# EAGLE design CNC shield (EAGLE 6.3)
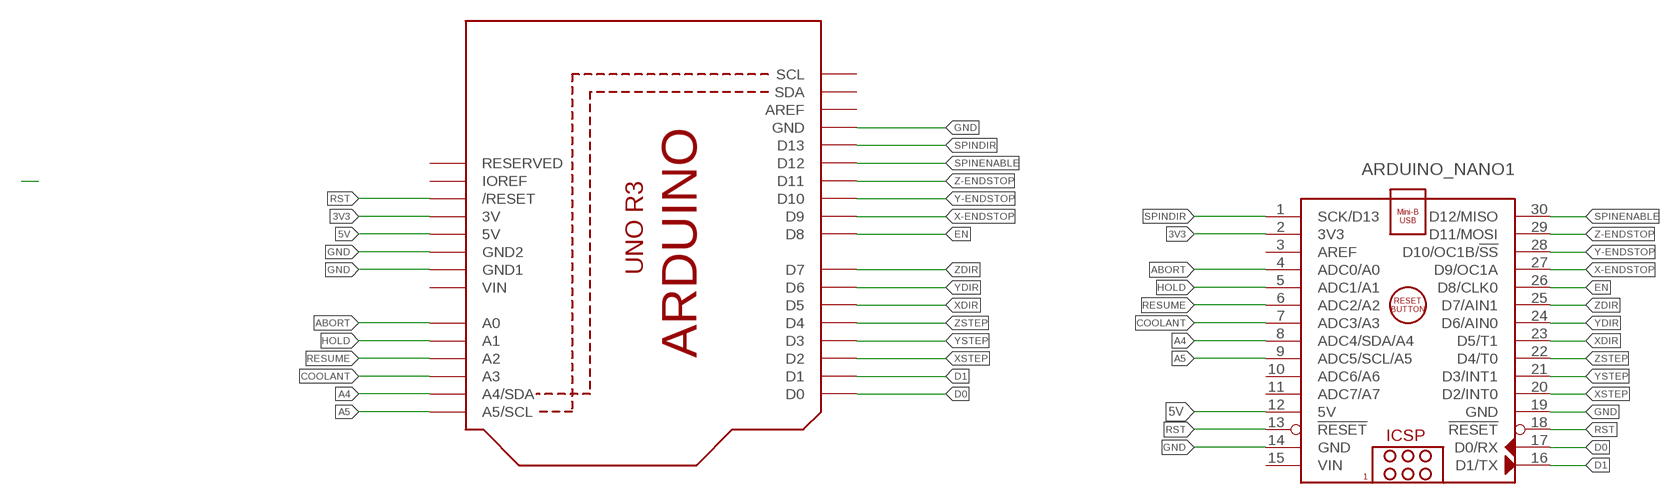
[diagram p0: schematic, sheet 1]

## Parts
ARDUINO_NANO1  ARDUINO_NANO  [ARDUINO_NANO]
U1  ARDUINOR3-BPLACE  [ARDUINOR3-BPLACE]

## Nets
3V3: ARDUINO_NANO1.2(3V3) U1.3V
5V: ARDUINO_NANO1.12(5V) U1.5V
A4: ARDUINO_NANO1.8(ADC4/SDA/A4) U1.A4(A4/SDA)
A5: ARDUINO_NANO1.9(ADC5/SCL/A5) U1.A5(A5/SCL)
ABORT: ARDUINO_NANO1.4(ADC0/A0) U1.A0
COOLANT: ARDUINO_NANO1.7(ADC3/A3) U1.A3
D0: ARDUINO_NANO1.17(D0/RX) U1.D0
D1: ARDUINO_NANO1.16(D1/TX) U1.D1
EN: ARDUINO_NANO1.26(D8/CLK0) U1.D8
GND: ARDUINO_NANO1.14(GND) ARDUINO_NANO1.19(GND) U1.GND U1.GND1 U1.GND2
HOLD: ARDUINO_NANO1.5(ADC1/A1) U1.A1
RESUME: ARDUINO_NANO1.6(ADC2/A2) U1.A2
RST: ARDUINO_NANO1.13(!RESET) ARDUINO_NANO1.18(!RESET) U1.RESET(/RESET)
SPINDIR: ARDUINO_NANO1.1(SCK/D13) U1.D13
SPINENABLE: ARDUINO_NANO1.30(D12/MISO) U1.D12
X-ENDSTOP: ARDUINO_NANO1.27(D9/OC1A) U1.D9
XDIR: ARDUINO_NANO1.23(D5/T1) U1.D5
XSTEP: ARDUINO_NANO1.20(D2/INT0) U1.D2
Y-ENDSTOP: ARDUINO_NANO1.28(D10/OC1B/!SS) U1.D10
YDIR: ARDUINO_NANO1.24(D6/AIN0) U1.D6
YSTEP: ARDUINO_NANO1.21(D3/INT1) U1.D3
Z-ENDSTOP: ARDUINO_NANO1.29(D11/MOSI) U1.D11
ZDIR: ARDUINO_NANO1.25(D7/AIN1) U1.D7
ZSTEP: ARDUINO_NANO1.22(D4/T0) U1.D4
Unconnected: ARDUINO_NANO1.3(AREF) ARDUINO_NANO1.10(ADC6/A6) ARDUINO_NANO1.11(ADC7/A7) U1.AREF U1.IOREF U1.RESERVED U1.SCL U1.SDA

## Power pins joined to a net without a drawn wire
VIN: ARDUINO_NANO1.15(VIN) U1.VIN

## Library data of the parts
ARDUINO_NANO1 = ArduinoNanoV30:ARDUINO_NANO: Arduino Nano V3.0 Module Overview: The Arduino Nano is a small, complete, and breadboard-friendly board based on the ATmega328 (Arduino Nano 3.x) or ATmega168 (Arduino Nano 2.x). It has more or less the same functionality of the Arduino Duemilanove, but in a different package. It lacks only a DC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
U1 = adafruit:ARDUINOR3: This is a new object for the new Arduino R3 - with extra pins that you may want to use (such as IOref, and duplicated A4/A5

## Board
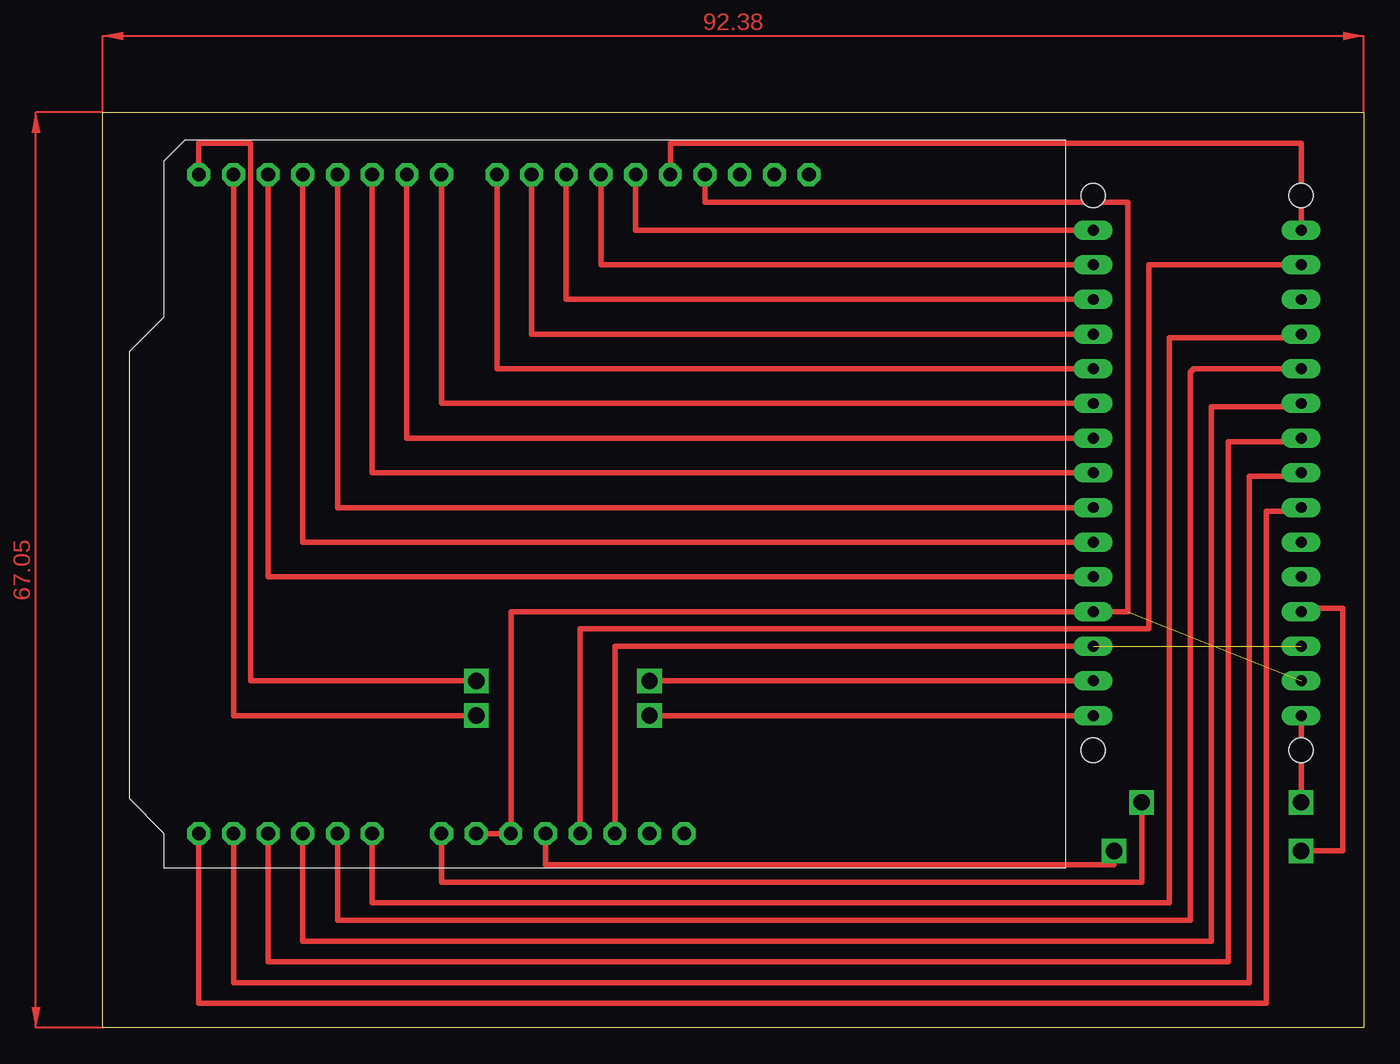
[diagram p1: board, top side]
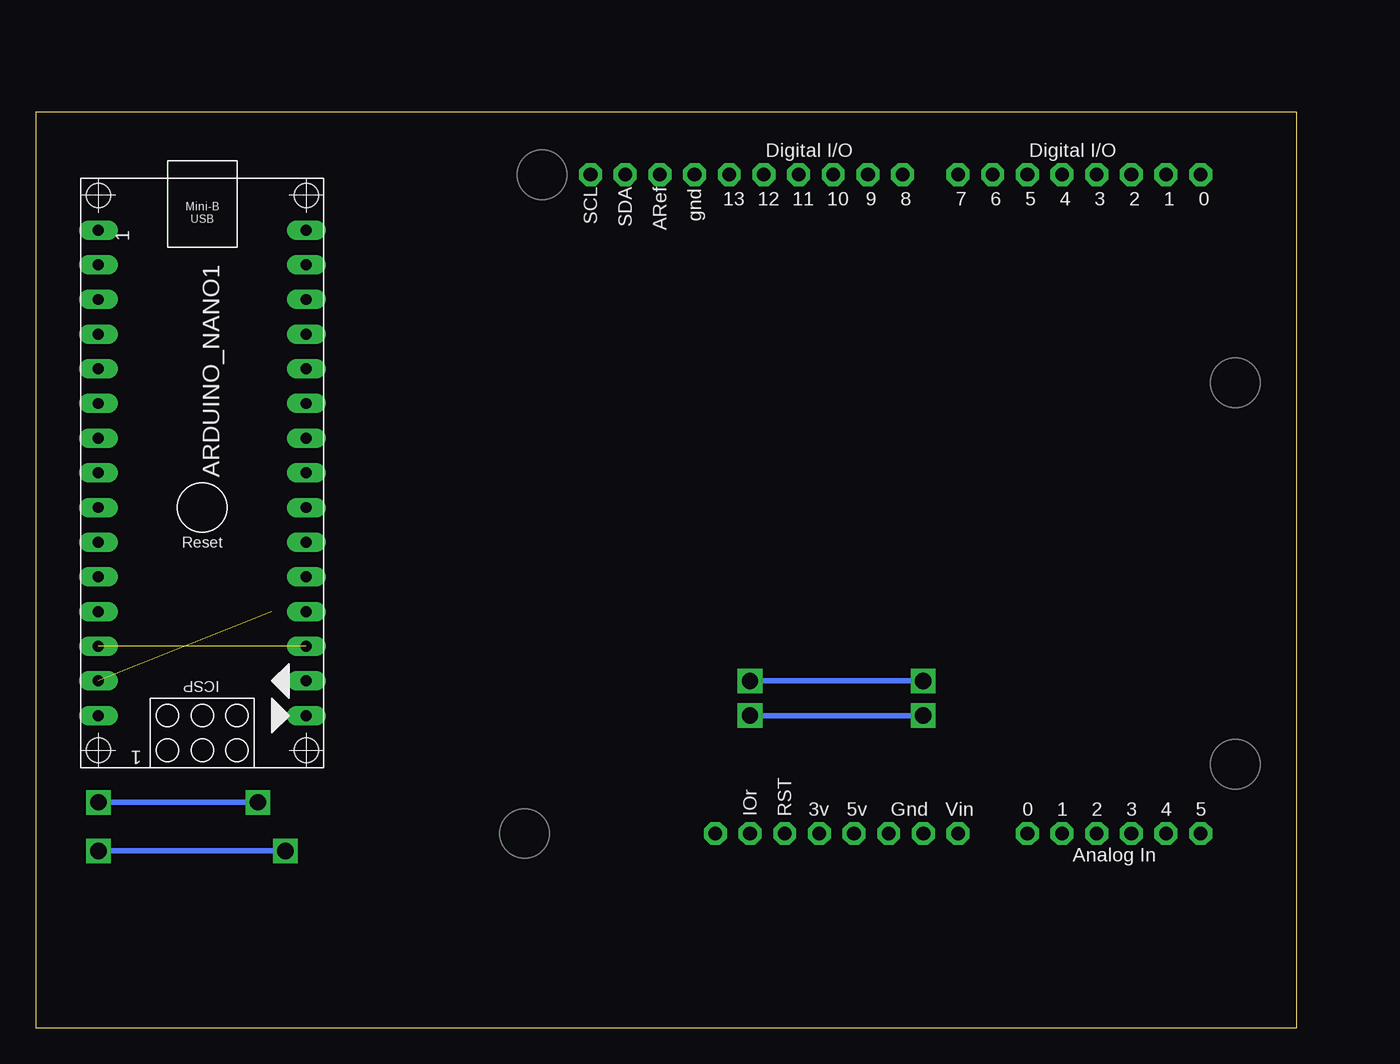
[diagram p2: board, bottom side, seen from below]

Size 92.38 x 67.05 mm. Coordinates in mm from the lower left corner, seen from the top.
Outline: 92.38,0 0,0 0,67.05 92.38,67.05 92.38,0
Copper layers (1*16): Top 0.035mm / dielectric 1.5mm / Bottom 0.035mm
Design rules "default": minimum track width 10mil, minimum drill 24mil, track to track 8mil, track to pad 8mil, pad to pad 8mil, via to via 8mil, smd to smd 8mil, copper to edge 40mil, drill to drill 8mil, minimum pad ring 10mil, minimum via ring 8mil, stop-mask expansion 4mil, vias tented up to drill 0mil, thermal gap 10mil

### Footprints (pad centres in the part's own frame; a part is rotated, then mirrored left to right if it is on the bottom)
ARDUINO_NANO = drill 0.8 pad 1.422 long: 1 -20.32,-7.62; 2 -17.78,-7.62; 3 -15.24,-7.62; 4 -12.7,-7.62; 5 -10.16,-7.62; 6 -7.62,-7.62; 7 -5.08,-7.62; 8 -2.54,-7.62; 9 0,-7.62; 10 2.54,-7.62; 11 5.08,-7.62; 12 7.62,-7.62; 13 10.16,-7.62; 14 12.7,-7.62; 15 15.24,-7.62; 16 15.24,7.62; 17 12.7,7.62; 18 10.16,7.62; 19 7.62,7.62; 20 5.08,7.62; 21 2.54,7.62; 22 0,7.62; 23 -2.54,7.62; 24 -5.08,7.62; 25 -7.62,7.62; 26 -10.16,7.62; 27 -12.7,7.62; 28 -15.24,7.62; 29 -17.78,7.62; 30 -20.32,7.62 | hole 1.778: -22.86,-7.62; -22.86,7.62; 17.78,7.62; 17.78,-7.62
ARDUINOR3-BPLACE = drill 1 pad 1.676 octagon: 3V 35.56,2.54; 5V 38.1,2.54; A0 50.8,2.54; A1 53.34,2.54; A2 55.88,2.54; A3 58.42,2.54; A4 60.96,2.54; A5 63.5,2.54; AREF 23.876,50.8; D0 63.5,50.8; D1 60.96,50.8; D2 58.42,50.8; D3 55.88,50.8; D4 53.34,50.8; D5 50.8,50.8; D6 48.26,50.8; D7 45.72,50.8; D8 41.656,50.8; D9 39.116,50.8; D10 36.576,50.8; D11 34.036,50.8; D12 31.496,50.8; D13 28.956,50.8; GND 26.416,50.8; GND1 43.18,2.54; GND2 40.64,2.54; IOREF 30.48,2.54; RESERVED 27.94,2.54; RESET 33.02,2.54; SCL 18.796,50.8; SDA 21.336,50.8; VIN 45.72,2.54

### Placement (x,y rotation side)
ARDUINO_NANO1  80.19,38.1 270 bottom
U1  70.54,11.68 0 bottom

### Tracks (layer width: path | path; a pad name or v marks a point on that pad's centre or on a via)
3V3
  Top 0.406: ARDUINO_NANO1.2 76.63,55.88 76.63,29.21 34.98,29.21 U1.3V
5V  (via drill 1.2)
  Top 0.406: U1.5V 32.44,11.94 74.09,11.94 v74.09,12.95 | v87.81,12.95 90.86,12.95 90.86,30.73 87.81,30.73 ARDUINO_NANO1.12
  Bottom 0.406: v74.09,12.95 v87.81,12.95
A4
  Top 0.406: U1.A4 9.58,3.3 84,3.3 84,40.39 87.81,40.39 ARDUINO_NANO1.8
A5
  Top 0.406: U1.A5 7.04,1.78 85.27,1.78 85.27,37.85 87.81,37.85 ARDUINO_NANO1.9
ABORT
  Top 0.406: U1.A0 19.74,9.14 78.16,9.14 78.16,50.55 87.81,50.55 ARDUINO_NANO1.4
COOLANT
  Top 0.406: U1.A3 12.12,4.83 82.47,4.83 82.47,42.93 87.81,42.93 ARDUINO_NANO1.7
D0  (via drill 0.6, 0.8, 1.2)
  Top 0.406: ARDUINO_NANO1.17 v40.06,25.4 | v27.36,25.4 10.85,25.4 10.85,64.77 7.04,64.77 U1.D0
  Bottom 0.406: v40.06,25.4 v27.36,25.4
D1  (via drill 0.6, 0.8, 1.2)
  Top 0.406: ARDUINO_NANO1.16 v40.06,22.86 | v27.36,22.86 9.58,22.86 U1.D1
  Bottom 0.406: v40.06,22.86 v27.36,22.86
EN
  Top 0.406: ARDUINO_NANO1.26 28.88,48.26 U1.D8
GND  (1 unrouted)
  Top 0.406: U1.GND 44.12,60.45 75.11,60.45 75.11,30.48 ARDUINO_NANO1.19 29.9,30.48 U1.GND2 U1.GND1
HOLD
  Top 0.406: U1.A1 17.2,7.87 79.68,7.87 79.68,48.01 79.93,48.26 ARDUINO_NANO1.5
RESUME
  Top 0.406: U1.A2 14.66,6.35 81.2,6.35 81.2,45.47 87.81,45.47 ARDUINO_NANO1.6
RST  (1 unrouted)
  Top 0.406: ARDUINO_NANO1.18 37.52,27.94 U1.RESET
SPINDIR
  Top 0.406: U1.D13 41.58,64.77 87.81,64.77 ARDUINO_NANO1.1
SPINENABLE
  Top 0.406: ARDUINO_NANO1.30 39.04,58.42 U1.D12
VIN  (via drill 1.2)
  Top 0.406: U1.VIN 24.82,10.67 76.12,10.67 v76.12,16.51 | v87.81,16.51 ARDUINO_NANO1.15
  Bottom 0.406: v76.12,16.51 v87.81,16.51
X-ENDSTOP
  Top 0.406: ARDUINO_NANO1.27 31.42,50.8 U1.D9
XDIR
  Top 0.406: ARDUINO_NANO1.23 19.74,40.64 U1.D5
XSTEP
  Top 0.406: ARDUINO_NANO1.20 12.12,33.02 U1.D2
Y-ENDSTOP
  Top 0.406: ARDUINO_NANO1.28 33.96,53.34 U1.D10
YDIR
  Top 0.406: ARDUINO_NANO1.24 22.28,43.18 U1.D6
YSTEP
  Top 0.406: ARDUINO_NANO1.21 14.66,35.56 U1.D3
Z-ENDSTOP
  Top 0.406: ARDUINO_NANO1.29 36.5,55.88 U1.D11
ZDIR
  Top 0.406: ARDUINO_NANO1.25 24.82,45.72 U1.D7
ZSTEP
  Top 0.406: ARDUINO_NANO1.22 17.2,38.1 U1.D4
(copper drawn outside any net)
  shapes: Top area x2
